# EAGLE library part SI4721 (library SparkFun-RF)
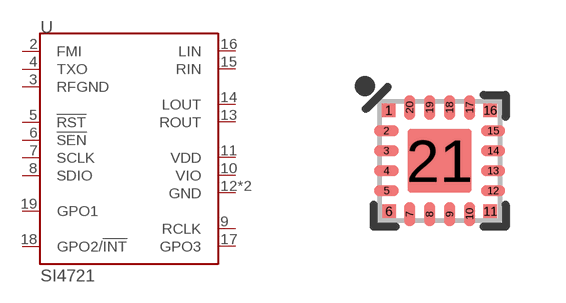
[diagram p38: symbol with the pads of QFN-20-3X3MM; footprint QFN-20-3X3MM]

Designator prefix U

## SI4721  [QFN-20-3X3MM]
2  FMI  in
3  RFGND  pwr
4  TXO
5  !RST  in
6  !SEN  in
7  SCLK  in
8  SDIO
9  RCLK  in
10  VIO  pwr
11  VDD  pwr
12  GND  pwr
13  ROUT  out
14  LOUT  out
15  RIN  in
16  LIN  in
17  GPO3  out
18  GPO2/!INT  out
19  GPO1  out
21  GND  pwr

## Footprint QFN-20-3X3MM (pad centres in mm)
20-Pin QFN Package 3 x 3 mm Used by Silicon Labs Si470x (Si4703, Si4707, etc.) FM Recievier Example Datasheet
smd 0.34 x 0.34: 1 -1.275,1.265; 6 -1.265,-1.265; 11 1.265,-1.265; 16 1.265,1.265
smd 0.61 x 0.28: 2 -1.335,0.75; 3 -1.335,0.25; 4 -1.335,-0.25; 5 -1.335,-0.75; 12 1.335,-0.75; 13 1.335,-0.25; 14 1.335,0.25; 15 1.335,0.75
smd 0.28 x 0.61: 7 -0.75,-1.335; 8 -0.25,-1.335; 9 0.25,-1.335; 10 0.75,-1.335; 17 0.75,1.335; 18 0.25,1.335; 19 -0.25,1.335; 20 -0.75,1.335
smd 1.6 x 1.6: 21 0,0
